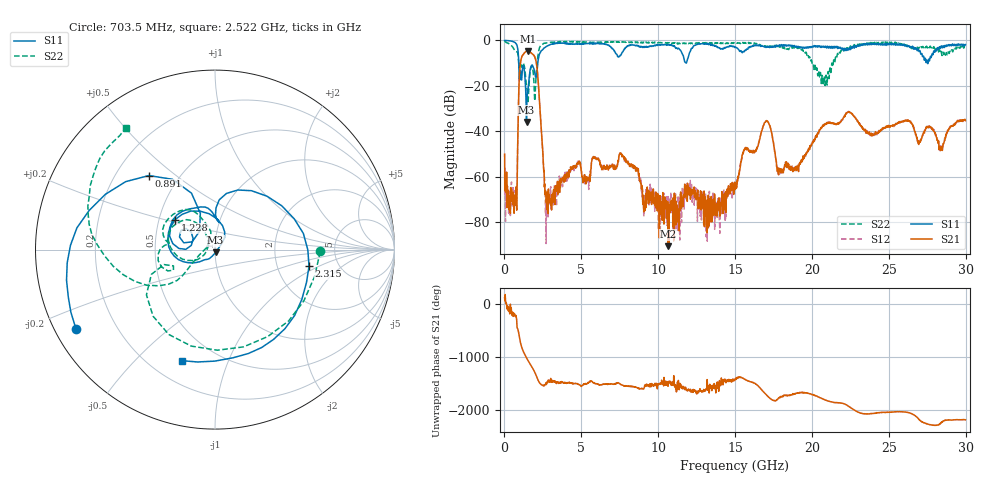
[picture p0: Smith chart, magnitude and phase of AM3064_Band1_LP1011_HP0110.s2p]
# Hz S DB R 50.0
!freq dBS11 angS11 dBS21 angS21 dBS12 angS12 dBS22 angS22
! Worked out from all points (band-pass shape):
!   1600 points, 10 MHz to 29.98 GHz, reference 50 ohm
!   highest |S21| = -4.64 dB at 1.51 GHz (marker M1); lowest = -90.6 dB at 10.64 GHz (marker M2)
!   |S21| within 3 dB of the highest: 1.107 GHz to 1.99 GHz (883.1 MHz wide, 57 % of centre)
!   lowest |S11| = -35.9 dB at 1.435 GHz (marker M3), VSWR 1.03, Z = 50.3 - j1.57 ohm
!   |S11| at or under -10 dB: 931.6 MHz to 2.164 GHz (1.233 GHz wide, 79.6 % of centre); 11.79775 GHz to 11.82628 GHz (28.53 MHz wide, 0.241 % of centre); 27.52146 GHz to 27.54942 GHz (27.95 MHz wide, 0.102 % of centre)
!   |S22| runs from -27.6 to -0.3 dB; largest |S21 - S12| = 0.009
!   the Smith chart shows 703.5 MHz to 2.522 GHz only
!   S11 on the Smith chart (normalised r, x): 703.5 MHz: 0.06, -0.26; 891 MHz: 0.34, +0.40; 1.228 GHz: 0.60, +0.22; 2.315 GHz: 3.05, -0.79; 2.522 GHz: 0.33, -0.69
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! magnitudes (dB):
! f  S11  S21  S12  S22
! 10 MHz  0.0  -50.1  -59.0  -0.3
! 703.5 MHz  -1.0  -68.5  -68.1  -4.6
! 891 MHz  -5.1  -35.2  -35.0  -6.8
! 1.041 GHz  -13.3  -9.9  -9.9  -9.9
! 1.228 GHz  -11.1  -6.2  -6.1  -10.1
! 1.435 GHz  -35.9  -4.7  -4.7  -19.8
! 1.51 GHz  -22.9  -4.6  -4.6  -26.3
! 2.016 GHz  -15.9  -8.2  -8.0  -20.8
! 2.315 GHz  -5.5  -30.7  -30.6  -2.7
! 2.522 GHz  -3.8  -53.5  -52.4  -1.5
! 2.803 GHz  -2.4  -68.9  -66.3  -1.0
! 5.015 GHz  -1.4  -57.7  -58.7  -0.6
! 7.62 GHz  -5.8  -50.1  -50.3  -0.7
! 10 GHz  -2.0  -74.8  -70.6  -1.0
! 10.64 GHz  -1.8  -90.6  -78.5  -1.2
! 15 GHz  -2.9  -65.6  -64.4  -1.3
! 17.01 GHz  -3.1  -35.5  -35.6  -2.6
! 17.93 GHz  -2.1  -57.6  -58.0  -2.4
! 19.99 GHz  -3.1  -45.9  -45.7  -9.3
! 25 GHz  -1.4  -38.0  -37.7  -1.1
! 28.41 GHz  -2.5  -47.5  -48.0  -5.1
! 29.98 GHz  -1.9  -35.3  -35.0  -3.1
